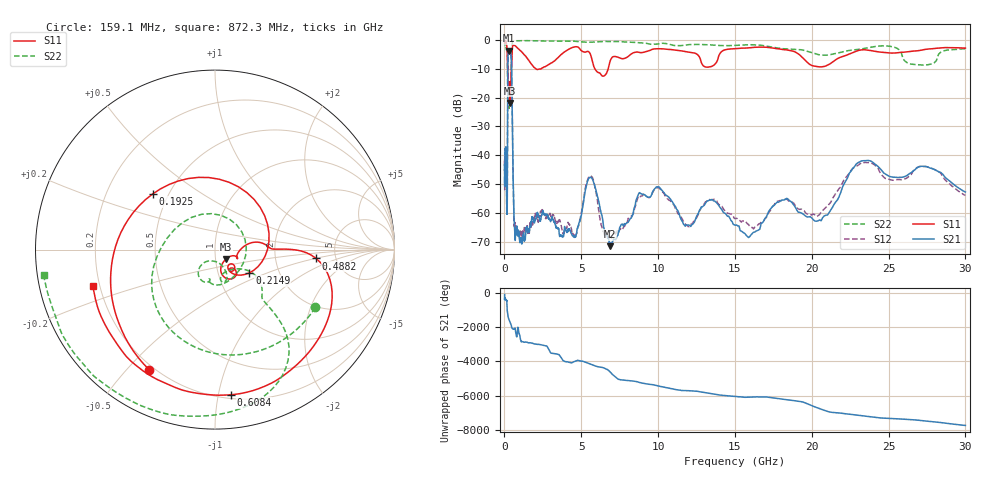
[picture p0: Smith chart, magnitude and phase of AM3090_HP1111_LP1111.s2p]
! Date/Time: Thu, Feb 28, 2019 2:10 PM
! Network Analyzer: Agilent Technologies E8364B Rev: A.07.50.67
! Sweep from 0.010 to 30.000 GHz, 1601 Points, Sweep Type: LOG
! Power Supply: 5.022 V, 0.002 A
# Hz S DB R 50
!freq MagS11 AngS11 MagS21 AngS21 MagS12 AngS12 MagS22 AngS22
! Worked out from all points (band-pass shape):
!   1601 points, 10 MHz to 30 GHz, reference 50 ohm
!   highest |S21| = -3.74 dB at 309.6 MHz (marker M1); lowest = -71.5 dB at 6.89 GHz (marker M2)
!   |S21| within 3 dB of the highest: 223.3 MHz to 447.6 MHz (224.3 MHz wide, 66.9 % of centre)
!   lowest |S11| = -21.9 dB at 354.4 MHz (marker M3), VSWR 1.18, Z = 55.9 - j6.17 ohm
!   |S11| at or under -10 dB: 207.3 MHz to 451.4 MHz (244.1 MHz wide, 74.1 % of centre); 2.037 GHz to 2.389 GHz (352.1 MHz wide, 15.9 % of centre); 5.883 GHz to 6.753 GHz (870.8 MHz wide, 13.8 % of centre)
!   |S22| runs from -23.7 to -0.2 dB; largest |S21 - S12| = 0.015
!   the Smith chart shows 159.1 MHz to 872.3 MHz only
!   S11 on the Smith chart (normalised r, x): 159.1 MHz: 0.18, -0.58; 192.5 MHz: 0.41, +0.32; 214.9 MHz: 1.41, -0.39; 488.2 MHz: 3.52, -0.51; 608.4 MHz: 0.23, -1.09; 872.3 MHz: 0.17, -0.14
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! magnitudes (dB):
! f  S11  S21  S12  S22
! 10 MHz  -0.3  -45.2  -43.3  -0.8
! 38.04 MHz  -0.2  -41.0  -41.5  -1.5
! 99.43 MHz  -0.9  -39.4  -38.7  -2.8
! 144.7 MHz  -1.7  -56.1  -59.0  -3.6
! 159.1 MHz  -2.3  -59.7  -55.8  -3.8
! 192.5 MHz  -6.6  -42.6  -42.0  -8.4
! 214.9 MHz  -12.7  -9.5  -9.4  -14.2
! 309.6 MHz  -14.5  -3.7  -3.7  -22.5
! 354.4 MHz  -21.9  -3.9  -3.9  -15.5
! 488.2 MHz  -5.0  -18.1  -18.0  -3.0
! 550.5 MHz  -2.0  -43.4  -43.6  -0.5
! 608.4 MHz  -1.8  -58.4  -60.0  -0.3
! 872.3 MHz  -3.0  -67.7  -66.5  -0.3
! 2.084 GHz  -10.2  -61.0  -61.1  -0.3
! 4.525 GHz  -2.5  -67.7  -67.5  -0.5
! 5.612 GHz  -5.2  -47.7  -47.0  -0.8
! 6.89 GHz  -7.2  -71.5  -68.9  -0.6
! 7.926 GHz  -6.2  -63.6  -63.9  -0.8
! 10.03 GHz  -3.1  -50.9  -51.3  -1.4
! 15.97 GHz  -2.8  -68.1  -64.7  -1.7
! 23.36 GHz  -3.4  -41.9  -42.6  -3.0
! 30 GHz  -2.9  -52.7  -53.9  -3.1
